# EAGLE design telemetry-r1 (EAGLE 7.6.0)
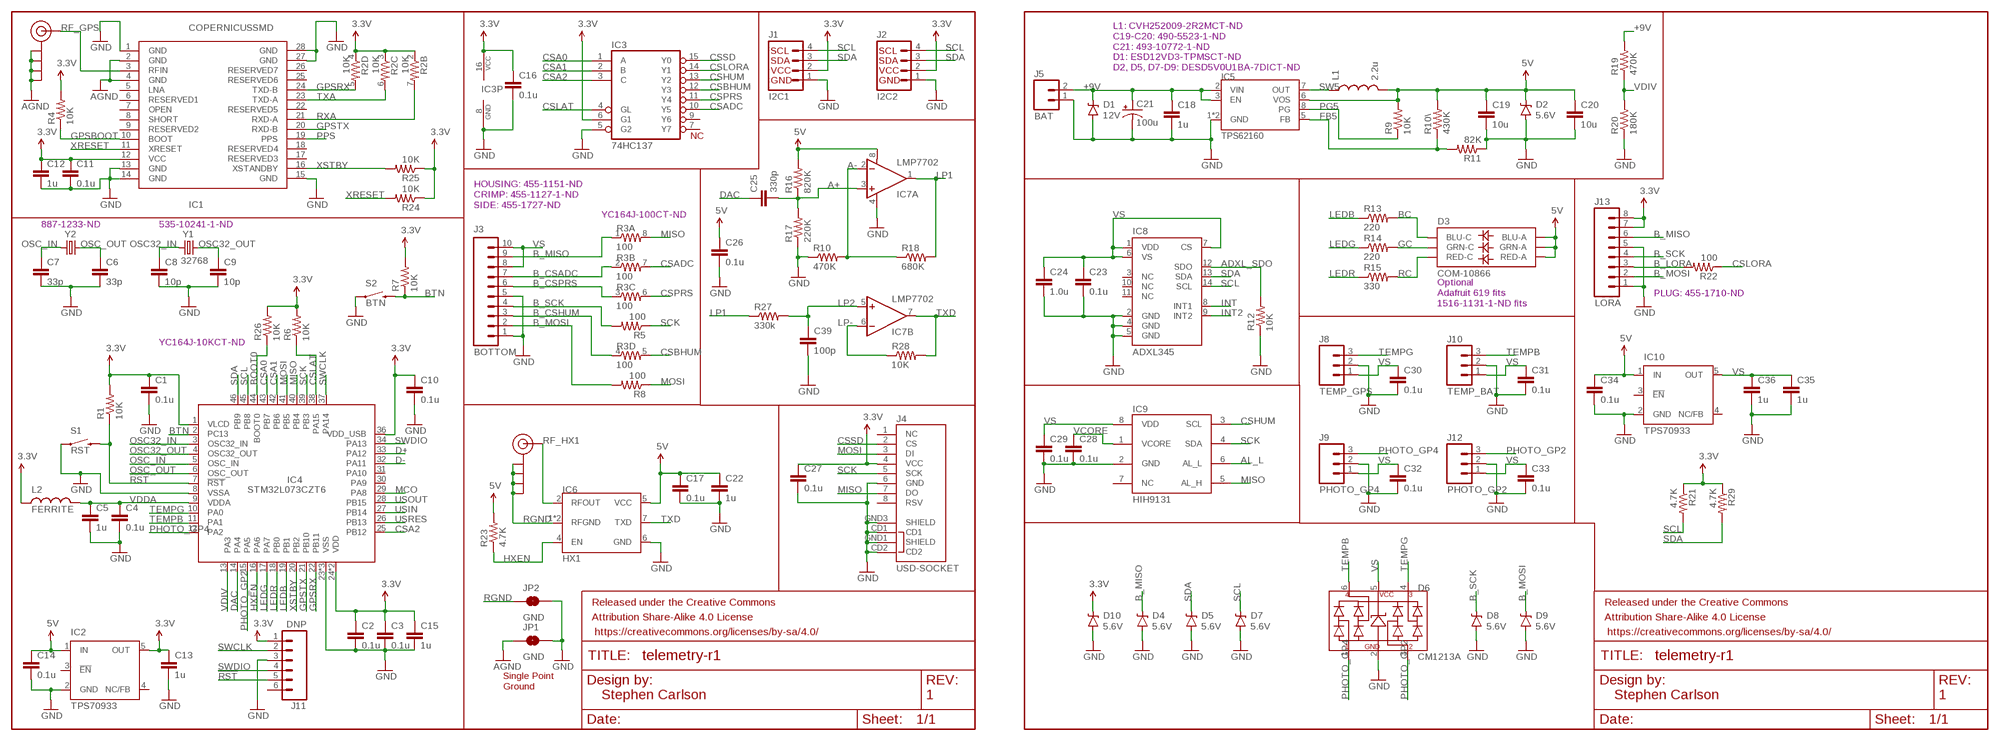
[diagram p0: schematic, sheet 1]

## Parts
C1  0.1u  CAP0805  [0805]
C2  0.1u  CAP0805  [0805]
C3  0.1u  CAP0805  [0805]
C4  0.1u  CAP0805  [0805]
C5  1u  CAP0805  [0805]
C6  33p  CAP0805  [0805]
C7  33p  CAP0805  [0805]
C8  10p  CAP0805  [0805]
C9  10p  CAP0805  [0805]
C10  0.1u  CAP0805  [0805]
C11  0.1u  CAP0805  [0805]
C12  1u  CAP0805  [0805]
C13  1u  CAP0805  [0805]
C14  0.1u  CAP0805  [0805]
C15  1u  CAP0805  [0805]
C16  0.1u  CAP0805  [0805]
C17  0.1u  CAP0805  [0805]
C18  1u  CAP0805  [0805]
C19  10u  CAP0805  [0805]
C20  10u  CAP0805  [0805]
C21  100u  CAP_POLPTH2  [CPOL-RADIAL-10UF-25V]
C22  1u  CAP0805  [0805]
C23  0.1u  CAP0805  [0805]
C24  1.0u  CAP0805  [0805]
C25  330p  CAP0805  [0805]
C26  0.1u  CAP0805  [0805]
C27  0.1u  CAP0805  [0805]
C28  0.1u  CAP0805  [0805]
C29  0.1u  CAP0805  [0805]
C30  0.1u  CAP0805  [0805]
C31  0.1u  CAP0805  [0805]
C32  0.1u  CAP0805  [0805]
C33  0.1u  CAP0805  [0805]
C34  0.1u  CAP0805  [0805]
C35  1u  CAP0805  [0805]
C36  1u  CAP0805  [0805]
C39  100p  CAP0805  [0805]
D1  12V  DIODE-ZENER5.6V  [SOD-323]
D2  5.6V  DIODE-ZENER5.6V  [SOD-323]
D3  COM-10866  LED-TRICOLOR-5050NO_IC  [LED-TRICOLOR-5050]
D4  5.6V  DIODE-ZENER5.6V  [SOD-323]
D5  5.6V  DIODE-ZENER5.6V  [SOD-323]
D6  CM1213A  [SC70-6L]
D7  5.6V  DIODE-ZENER5.6V  [SOD-323]
D8  5.6V  DIODE-ZENER5.6V  [SOD-323]
D9  5.6V  DIODE-ZENER5.6V  [SOD-323]
D10  5.6V  DIODE-ZENER5.6V  [SOD-323]
FRAME1  FRAME-LETTERNO_PACKAGE  [DUMMY]
FRAME2  FRAME-LETTERNO_PACKAGE  [DUMMY]
IC1  COPERNICUSSMD  [COPERNICUS]
IC2  TPS70933  TPS77033  [SOT23-DBV]
IC3  74HC137  74LS137PW  [TSSOP16]
IC4  STM32L073CZT6  STM32L07C  [TQFP48]
IC5  TPS62160  [MSOP8]
IC6  HX1  [HX1]
IC7  LMP7702  OPAMP-DUALU  [SO08]
IC8  ADXL345  [LGA14]
IC9  HIH9131  HIH6131  [SOIC8]
IC10  TPS70933  TPS77033  [SOT23-DBV]
J1  I2C1  I2C_STANDARD_NO_SILK  [1X04_NO_SILK]
J2  I2C2  I2C_STANDARD_NO_SILK  [1X04_NO_SILK]
J3  BOTTOM  M102MM  [1X10-2MM]
J4  USD-SOCKET  [MICROSD_1:1]
J5  BAT  M02PTH  [1X02]
J6  SMA_EDGE  [SMA-EDGE]
J7  SMA_EDGE  [SMA-EDGE]
J8  TEMP_GPS  M03JST-PTH  [JST-3-PTH]
J9  PHOTO_GP4  M03JST-PTH  [JST-3-PTH]
J10  TEMP_BAT  M03JST-PTH  [JST-3-PTH]
J11  DNP  M06LOCK  [1X06_LOCK]
J12  PHOTO_GP2  M03JST-PTH  [JST-3-PTH]
J13  LORA  1X08  [1X08-2MM]
JP1  GND  JUMPER-PAD-2-NC_BY_TRACE  [PAD-JUMPER-2-NC_BY_TRACE_YES_SILK]
JP2  GND  JUMPER-PAD-2-NC_BY_TRACE  [PAD-JUMPER-2-NC_BY_TRACE_YES_SILK]
L1  2.2u  INDUCTOR1008  [1008]
L2  FERRITE  INDUCTOR1206  [1206]
R1  10K  RESISTOR0805-RES  [0805]
R2  10K  RESISTOR-ARRAY0603-ARV  [0603-ARV]
R3  100  RESISTOR-ARRAY0603-ARV  [0603-ARV]
R4  10K  RESISTOR0805-RES  [0805]
R5  100  RESISTOR0805-RES  [0805]
R6  10K  RESISTOR0805-RES  [0805]
R7  10K  RESISTOR0805-RES  [0805]
R8  100  RESISTOR0805-RES  [0805]
R9  10K  RESISTOR0805-RES  [0805]
R10  470K  RESISTOR0805-RES  [0805]
R10\  430K  RESISTOR0805-RES  [0805]
R11  82K  RESISTOR0805-RES  [0805]
R12  10K  RESISTOR0805-RES  [0805]
R13  220  RESISTOR0805-RES  [0805]
R14  220  RESISTOR0805-RES  [0805]
R15  330  RESISTOR0805-RES  [0805]
R16  820K  RESISTOR0805-RES  [0805]
R17  220K  RESISTOR0805-RES  [0805]
R18  680K  RESISTOR0805-RES  [0805]
R19  470K  RESISTOR0805-RES  [0805]
R20  180K  RESISTOR0805-RES  [0805]
R21  4.7K  RESISTOR0805-RES  [0805]
R22  100  RESISTOR0805-RES  [0805]
R23  4.7K  RESISTOR0805-RES  [0805]
R24  10K  RESISTOR0805-RES  [0805]
R25  10K  RESISTOR0805-RES  [0805]
R26  10K  RESISTOR0805-RES  [0805]
R27  330k  RESISTOR0805-RES  [0805]
R28  10K  RESISTOR0805-RES  [0805]
R29  4.7K  RESISTOR0805-RES  [0805]
S1  RST  SWITCH  [TACTILE-PTH-THIN]
S2  BTN  SWITCH  [TACTILE-PTH-THIN]
Y1  32768  CRYSTAL  [ABS25]
Y2  8M  CRYSTALSMD  [HC49UP]

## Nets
3.3V: C1.1 C2.1 C3.1 C10.1 C11.1 C12.1 C13.1 C15.1 C16.1 C27.1 D10.C IC1.12(VCC) IC2.5(OUT) IC3.6(G1) IC3.16(VCC) IC4.1(VLCD) IC4.24(VDD) IC4.36(VDD_USB) IC4.48(VDD) J1.2 J2.2 J4.4(VCC) J11.1 J13.7 J13.8 L2.1 R1.2 R2.2 R2.3 R2.4 R4.2 R6.2 R7.2 R21.1 R24.1 R25.1 R26.2 R29.1
5V: C14.1 C17.1 C19.1 C20.1 C22.1 C26.1 C34.1 D2.C D3.1(GRN-A) D3.2(RED-A) D3.3(BLU-A) IC2.1(IN) IC5.6(VOS) IC6.5(VCC) IC7.8(A:V+) IC10.1(IN) L1.2 R9.2 R10\.2 R16.2 R23.2
!RST!: IC4.7(!RST!) J11.5 R1.1 S1.2
+9V: C18.1 C21.1(+) D1.C IC5.2(VIN) IC5.3(EN) J5.2 R19.2
A+: C25.2 IC7.3(A:+IN) R16.1 R17.2
A-: IC7.2(A:-IN) R10.2 R18.1
ADXL_SDO: IC8.12(SDO) R12.2
AGND: IC1.2(GND) IC1.4(GND) J7.GND@0(GND) J7.GND@1(GND) J7.GND@2(GND) J7.GND@3(GND) JP1.1
AL_L: IC9.6(AL_L)
B_CSADC: J3.7 R3.2
B_CSHUM: J3.3 R3.4
B_CSPRS: J3.6 R3.3
B_LORA: J13.3 R22.2
B_MISO: D4.C J3.9 J13.6 R3.1
B_MOSI: D9.C J3.2 J13.2 R8.2
B_SCK: D8.C J3.4 J13.4 R5.2
BC: D3.4(BLU-C) R13.2
BOOT0: IC4.44(BOOT0) R26.1
BTN: IC4.2(PC13) R7.1 S2.2
CSA0: IC3.1(A) IC4.43(PB7)
CSA1: IC3.2(B) IC4.42(PB6)
CSA2: IC3.3(C) IC4.25(PB12)
CSADC: IC3.10(Y5) R3.7
CSBHUM: IC3.12(Y3) R3.5
CSHUM: IC3.13(Y2) IC9.3(SCL)
CSLAT: IC3.4(GL) IC4.38(PA15) R6.1
CSLORA: IC3.14(Y1) R22.1
CSPRS: IC3.11(Y4) R3.6
CSSD: IC3.15(Y0) J4.2(CS)
D+: IC4.33(PA12)
D-: IC4.32(PA11)
DAC: C25.1 IC4.14(PA4)
FB5: IC5.5(FB) R10\.1 R11.2
GC: D3.6(GRN-C) R14.2
GND: C1.2 C2.2 C3.2 C4.2 C5.2 C6.2 C7.2 C8.2 C9.2 C10.2 C11.2 C12.2 C13.2 C14.2 C15.2 C16.2 C17.2 C18.2 C19.2 C20.2 C21.2(-) C22.2 C23.2 C24.2 C26.2 C27.2 C28.2 C29.2 C30.2 C31.2 C32.2 C33.2 C34.2 C35.2 C36.2 C39.2 D1.A D2.A D4.A D5.A D6.2(GND) D7.A D8.A D9.A D10.A IC1.1(GND) IC1.13(GND) IC1.14(GND) IC1.15(GND) IC1.27(GND) IC1.28(GND) IC2.2(GND) IC3.5(G2) IC3.8(GND) IC4.8(VSSA) IC4.23(VSS) IC4.35(VSS) IC4.47(VSS) IC5.1(GND) IC5.4(GND) IC6.6(GND) IC7.4(A:V-) IC8.2(GND) IC8.4(GND) IC8.5(GND) IC9.2(GND) IC10.2(GND) J1.1 J2.1 J3.1 J3.5 J4.6(GND) J4.CD1 J4.CD2 J4.GND1(SHIELD) J4.GND3(SHIELD) J5.1 J8.2 J9.2 J10.2 J11.3 J12.2 J13.1 J13.5 JP1.2 JP2.2 R10.1 R11.1 R12.1 R17.1 R20.1 S1.1 S2.1
GPSBOOT: IC1.10(BOOT) R4.1
GPSRX: IC1.24(TXD-B) IC4.22(PB11) R2.5
GPSTX: IC1.20(RXD-B) IC4.21(PB10)
HXEN: IC4.16(PA6) IC6.4(EN) R23.1
INT: IC8.8(INT1)
INT2: IC8.9(INT2)
LEDB: IC4.19(PB1) R13.1
LEDG: IC4.17(PA7) R14.1
LEDR: IC4.18(PB0) R15.1
LP1: IC7.1(A:OUT) R18.2 R27.1
LP2: C39.1 IC7.5(B:+IN) R27.2
LP-: IC7.6(B:-IN) R28.1
MCO: IC4.29(PA8)
MISO: IC4.40(PB4) IC9.5(AL_H) J4.7(DO) R3.8
MOSI: IC4.41(PB5) J4.3(DI) R8.1
OSC32_IN: C8.1 IC4.3(OSC32_IN) Y1.1
OSC32_OUT: C9.1 IC4.4(OSC32_OUT) Y1.4
OSC_IN: C7.1 IC4.5(OSC_IN) Y2.1
OSC_OUT: C6.1 IC4.6(OSC_OUT) Y2.2
PG5: IC5.8(PG) R9.1
PHOTO_GP2: D6.3(CH2) IC4.15(PA5) J12.3
PHOTO_GP4: D6.1(CH1) IC4.12(PA2) J9.3
PPS: IC1.19(PPS)
RC: D3.5(RED-C) R15.2
RF_GPS: IC1.3(RFIN) J7.SIG(SIGNAL)
RF_HX1: IC6.2(RFOUT) J6.SIG(SIGNAL)
RGND: IC6.1(RFGND) IC6.3(RFGND) J6.GND@0(GND) J6.GND@1(GND) J6.GND@2(GND) J6.GND@3(GND) JP2.1
RXA: IC1.21(RXD-A) R2.7
SCK: IC4.39(PB3) IC9.4(SDA) J4.5(SCK) R5.1
SCL: D7.C IC4.45(PB8) IC8.14(SCL) J1.4 J2.4 R21.2
SDA: D5.C IC4.46(PB9) IC8.13(SDA) J1.3 J2.3 R29.2
SW5: IC5.7(OUT) L1.1
SWCLK: IC4.37(PA14) J11.2
SWDIO: IC4.34(PA13) J11.4
TEMPB: D6.6(CH4) IC4.11(PA1) J10.3
TEMPG: D6.4(CH3) IC4.10(PA0) J8.3
TXA: IC1.23(TXD-A) R2.6
TXD: IC6.7(TXD) IC7.7(B:OUT) R28.2
USIN: IC4.27(PB14)
USOUT: IC4.28(PB15)
USRES: IC4.26(PB13)
VCORE: C28.1 IC9.1(VCORE)
VDDA: C4.1 C5.1 IC4.9(VDDA) L2.2
VDIV: IC4.13(PA3) R19.1 R20.2
VS: C23.1 C24.1 C29.1 C30.1 C31.1 C32.1 C33.1 C35.1 C36.1 D6.5(VCC) IC8.1(VDD) IC8.6(VS) IC8.7(CS) IC9.8(VDD) IC10.5(OUT) J3.8 J3.10 J8.1 J9.1 J10.1 J12.1
XRESET: IC1.11(XRESET) R24.2
XSTBY: IC1.16(XSTANDBY) IC4.20(PB2) R25.2
Unconnected: IC1.5(LNA) IC1.6(RESERVED1) IC1.7(OPEN) IC1.8(SHORT) IC1.9(RESERVED2) IC1.17(RESERVED3) IC1.18(RESERVED4) IC1.22(RESERVED5) IC1.25(RESERVED6) IC1.26(RESERVED7) IC2.3(!EN) IC2.4(NC/FB) IC3.7(Y7) IC3.9(Y6) IC4.30(PA9) IC4.31(PA10) IC8.3(NC) IC8.10(NC) IC8.11(NC) IC9.7(NC) IC10.3(!EN) IC10.4(NC/FB) J4.1(NC) J4.8(RSV) J11.6 R2.1 R2.8

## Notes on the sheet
- L1: CVH252009-2R2MCT-ND
  C19-C20: 490-5523-1-ND
  C21: 493-10772-1-ND
  D1: ESD12VD3-TPMSCT-ND
  D2, D5, D7-D9: DESD5V0U1BA-7DICT-ND
- NC
- HOUSING: 455-1151-ND
  CRIMP: 455-1127-1-ND
  SIDE: 455-1727-ND
- YC164J-100CT-ND
- 887-1233-ND | 535-10241-1-ND
- PLUG: 455-1710-ND
- Optional
  Adafruit 619 fits
  1516-1131-1-ND fits
- YC164J-10KCT-ND
- Single Point
  Ground
- Stephen Carlson | 1 | Stephen Carlson | 1

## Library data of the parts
C1-C20 C22-C36 C39 = SparkFun-Passives:CAP: Capacitor
C21 = SparkFun-Passives:CAP_POL: Capacitor Polarized
D1 = SparkFun-DiscreteSemi:DIODE-ZENER: Zener Diode; PROD_ID: DIO-12442; VALUE: 5.6V
D2 D4 D5 D7-D10 = SparkFun-DiscreteSemi:DIODE-ZENER: Zener Diode; PROD_ID: DIO-12442
D3 = SparkFun-LED:LED-TRICOLOR-5050
D6 = HAB:CM1213A: CM1213A CM1213A 4-channel ESD protection device
FRAME1 FRAME2 = SparkFun-Aesthetics:FRAME-LETTER: Schematic Frame; DESIGNER: Nobody; VERSION: v01
IC1 = SparkFun-RF:COPERNICUS: Copernicus II GPS- Trimble recommended layout and paste layer. Footprint production proven. Spark Fun Electronics SKU : GPS-07951
IC2 IC10 = texas:TPS770*: ULTRALOW-POWER 50-mA LOW-DROPOUT LINEAR REGULATORS 50-mA Low-Dropout Regulator Source: http://focus.ti.com/lit/ds/symlink/tps77001.pdf; MF: TEXAS INSTRUMENTS; MPN: TPS77033DBVT; OC_FARNELL: 8461570; OC_NEWARK: 77C1187
IC3 = HAB:74*137: 3-line to 8-line DECODER/DEMULTIPLEXER, address LATCH
IC4 = stm32xx:STM32L07*C: STM32L07XC STM32L07X series in LQFP-48 package
IC5 = HAB:TPS62160: TPS62160 Adjustable switch-mode D-CAP2 regulator
IC6 = HAB:HX1: Radiometrix HX1 High-power VHF Narrow Band 300 mW Transmitter
IC7 = SparkFun-AnalogIC:OPAMP-DUAL: Generic op-amp footprint
IC8 = SparkFun-Sensors:ADXL345: 3-axis SPI/I2C 2/4/8/16g accelerometer
IC9 = SparkFun-AnalogIC:HIH6131
J1 J2 = SparkFun-Connectors:I2C_STANDARD: SparkFun has standardized on a pinout for all I2C based sensor breakouts. This pinout allows I2C boards to be plugged directly into the headers on Arduino Uno compatible boards, and to be daisy chained easily.
J3 = SparkFun-Connectors:M10: Header 10 Standard 10-pin 0.1" header. Use with straight break away headers (SKU : PRT-00116), right angle break away headers (PRT-00553), swiss pins (PRT-00743), machine pins (PRT-00117), and female headers (PRT-00115).
J4 = SparkFun-Connectors:USD-SOCKET: microSD Socket Push-push type uSD socket. Schematic element and footprint production proven. Spark Fun Electronics SKU : PRT-00127. tDoc lines correctly indicate media card edge positions when inserting (unlocked, locked, depressed). NOTE: CD1 and CD2 are connected internally; PROD_ID: CONN-07820
J5 = SparkFun-Connectors:M02: Standard 2-pin 0.1" header. Use with
J6 J7 = SparkFun-Connectors:SMA_EDGE: SMA Antenna Connector End launch SMA connector. The paste layer has been removed so that the connector can be hand soldered onto the board after reflow.
J8-J10 J12 = SparkFun-Connectors:M03: Header 3 Standard 3-pin 0.1" header. Use with straight break away headers (SKU : PRT-00116), right angle break away headers (PRT-00553), swiss pins (PRT-00743), machine pins (PRT-00117), and female headers (PRT-00115). Molex polarized connector foot print use with SKU : PRT-08232 with associated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; SKU: PRT-09915
J11 = SparkFun-Connectors:M06: Header 6 Standard 6-pin 0.1" header. Use with straight break away headers (SKU : PRT-00116), right angle break away headers (PRT-00553), swiss pins (PRT-00743), machine pins (PRT-00117), and female headers (PRT-00115). Molex polarized connector foot print use with SKU : PRT-08094 with associated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
J13 = HAB:1X08: 1X08 1x8 header
JP1 JP2 = SparkFun-Passives:JUMPER-PAD-2-NC_BY_TRACE
L1 L2 = HAB:INDUCTOR: INDUCTOR
R1 R4-R10 R10\ R11-R29 = SparkFun-Passives:RESISTOR: Resistor
R2 R3 = SparkFun-Passives:RESISTOR-ARRAY: Array Chip Resistor Source: RS Component / Phycomp
S1 S2 = HAB:SWITCH: SWITCH
Y1 = HAB:CRYSTAL: CRYSTAL
Y2 = SparkFun-FreqCtrl:CRYSTAL: Various standard crystals. Proven footprints.

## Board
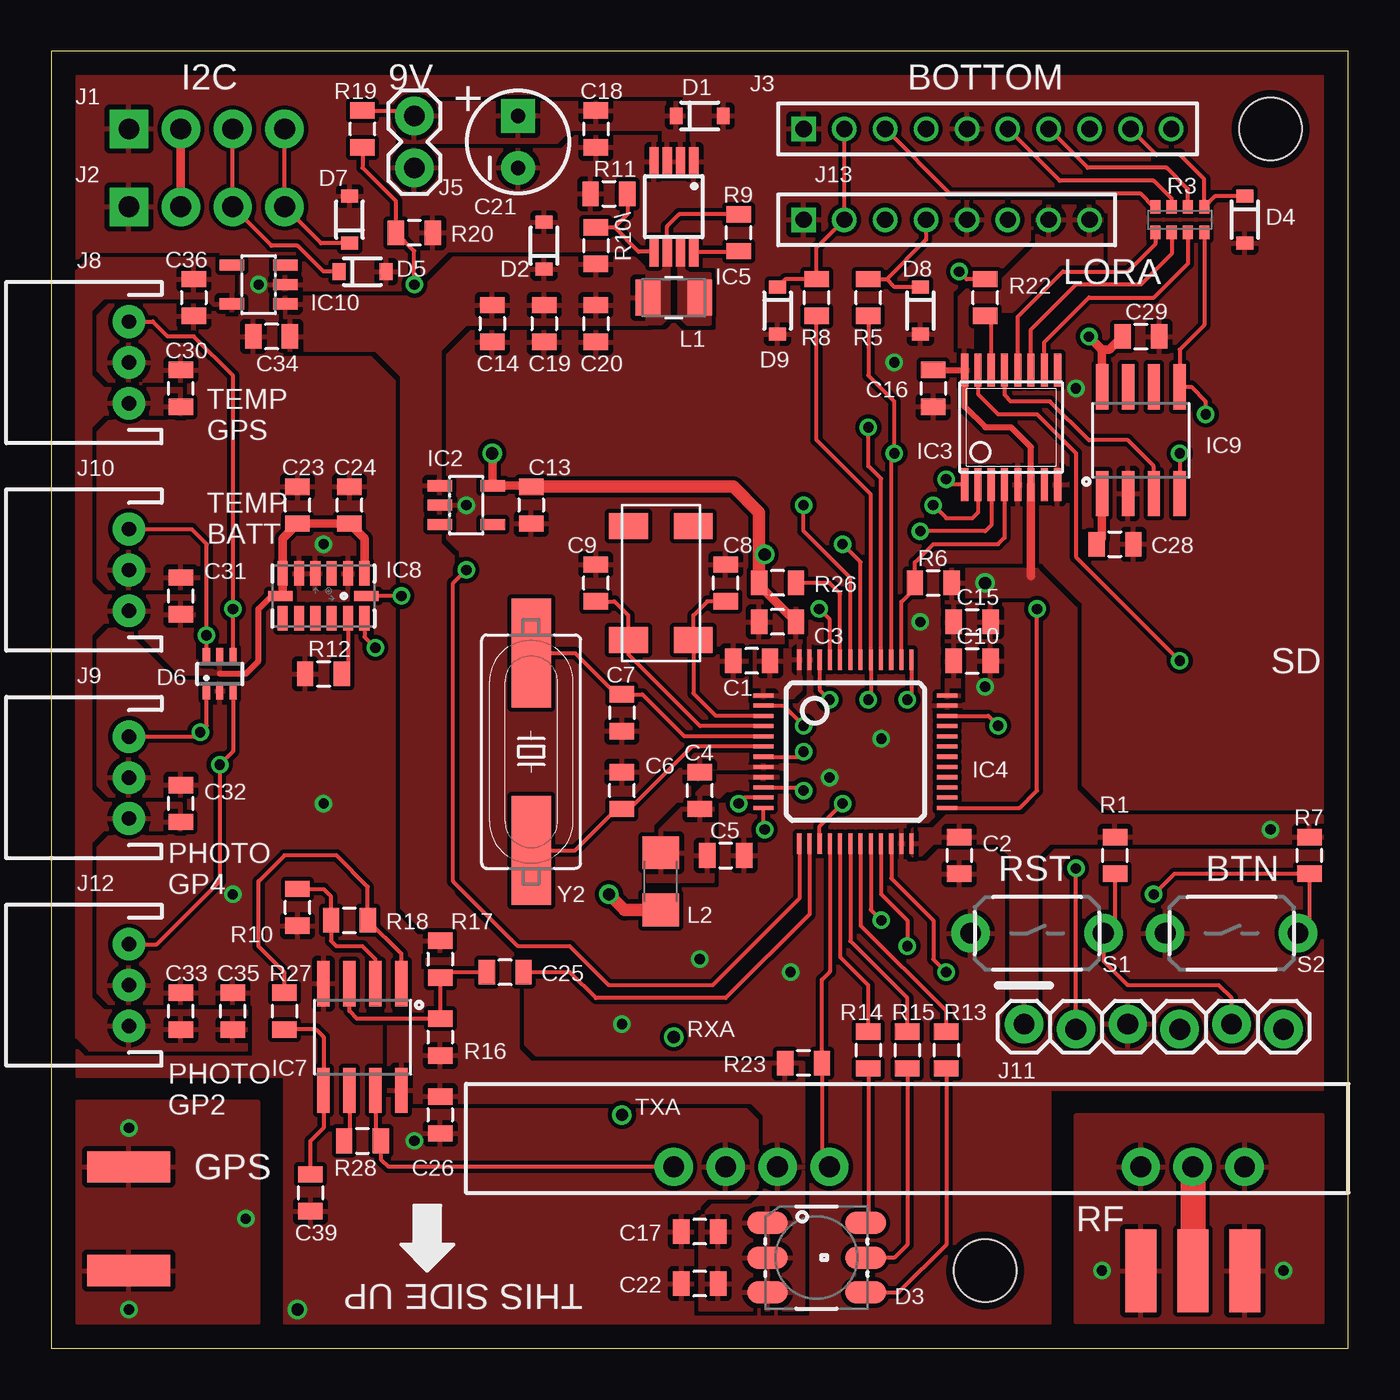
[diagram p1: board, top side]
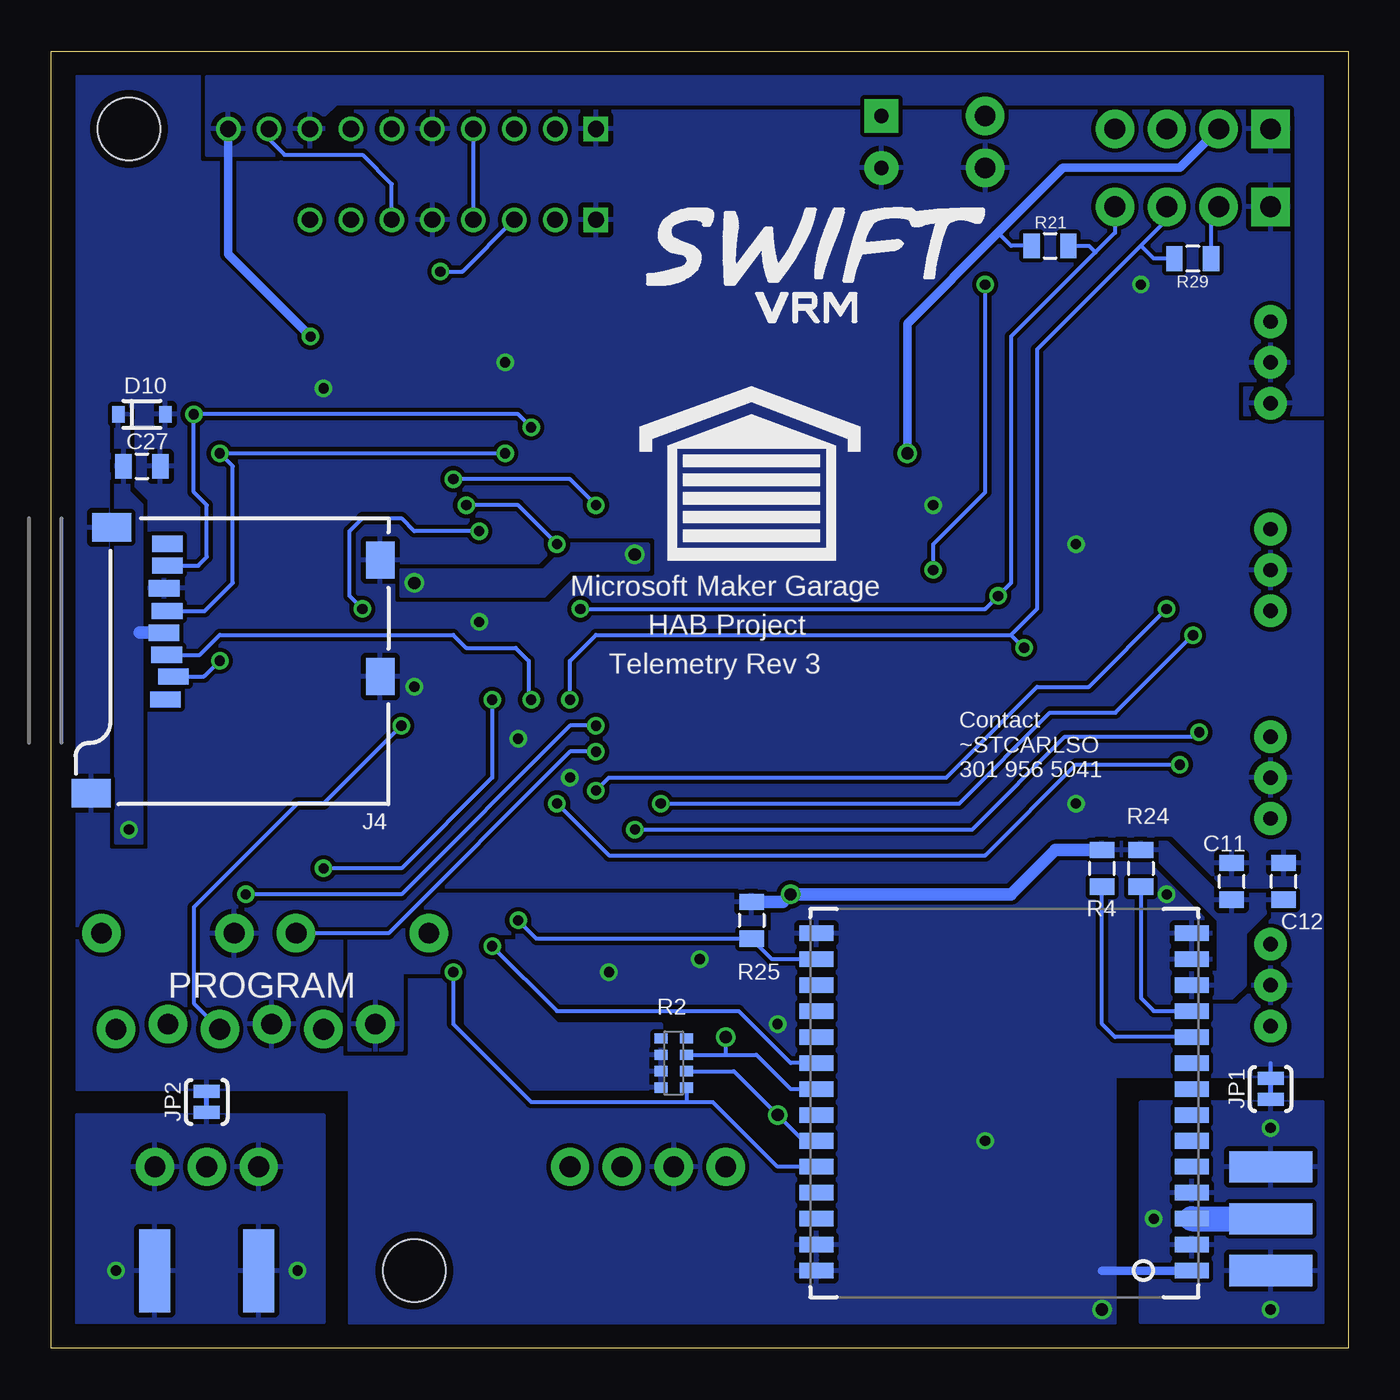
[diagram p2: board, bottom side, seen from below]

Size 63.5 x 63.5 mm. Coordinates in mm from the lower left corner, seen from the top.
Outline: 0,0 63.5,0 63.5,63.5 0,63.5 0,0
Copper layers (1*16): Top 0.0356mm / dielectric 1.5011mm / Bottom 0.0356mm
Design rules "LaenPCBOrder *": minimum track width 6mil, minimum drill 13mil, track to track 8mil, track to pad 8mil, pad to pad 8mil, via to via 8mil, smd to smd 6mil, copper to edge 15mil, drill to drill 6mil, minimum pad ring 7mil, minimum via ring 7mil, stop-mask expansion 3mil, vias tented up to drill 0mil, thermal gap 10mil
Holes 3.05 mm at 45.72,3.81 59.69,59.69

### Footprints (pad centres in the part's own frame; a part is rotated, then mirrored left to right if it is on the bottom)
0805 = smd 0.8 x 1.2: 1 -0.9,0; 2 0.9,0
CPOL-RADIAL-10UF-25V = drill 0.7 pad 1.651 square: 1 1.27,0 | drill 0.7 pad 1.651: 2 -1.27,0
SOD-323 = smd 0.63 x 0.83: A 1.15,0; C -1.15,0
LED-TRICOLOR-5050 = smd 2 x 1.1: 1 -2.4,1.7; 2 -2.4,0; 3 -2.4,-1.7; 4 2.4,-1.7; 5 2.4,0; 6 2.4,1.7
SC70-6L = smd 0.35 x 0.8: 1 -0.65,-0.85; 2 0,-0.85; 3 0.65,-0.85; 4 0.65,0.85; 5 0,0.85; 6 -0.65,0.85
COPERNICUS = smd 0.762 x 1.651: 1 0,-18.364; 2 1.27,-18.364; 3 2.54,-18.364; 4 3.81,-18.364; 5 5.08,-18.364; 6 6.35,-18.364; 7 7.62,-18.364; 8 8.89,-18.364; 9 10.16,-18.364; 10 11.43,-18.364; 11 12.7,-18.364; 12 13.97,-18.364; 13 15.24,-18.364; 14 16.51,-18.364; 15 16.51,0; 16 15.24,0; 17 13.97,0; 18 12.7,0; 19 11.43,0; 20 10.16,0; 21 8.89,0; 22 7.62,0; 23 6.35,0; 24 5.08,0; 25 3.81,0; 26 2.54,0; 27 1.27,0; 28 0,0
SOT23-DBV = smd 0.55 x 1.2: 1 -0.95,-1.3; 2 0,-1.3; 3 0.95,-1.3; 4 0.95,1.3; 5 -0.95,1.3
TSSOP16 = smd 0.35 x 1.6: 1 -2.275,-2.8; 2 -1.625,-2.8; 3 -0.975,-2.8; 4 -0.325,-2.8; 5 0.325,-2.8; 6 0.975,-2.8; 7 1.625,-2.8; 8 2.275,-2.8; 9 2.275,2.8; 10 1.625,2.8; 11 0.975,2.8; 12 0.325,2.8; 13 -0.325,2.8; 14 -0.975,2.8; 15 -1.625,2.8; 16 -2.275,2.8
TQFP48 = smd 0.2 x 1: 1 -2.75,-4.5; 2 -2.25,-4.5; 3 -1.75,-4.5; 4 -1.25,-4.5; 5 -0.75,-4.5; 6 -0.25,-4.5; 7 0.25,-4.5; 8 0.75,-4.5; 9 1.25,-4.5; 10 1.75,-4.5; 11 2.25,-4.5; 12 2.75,-4.5; 25 2.75,4.5; 26 2.25,4.5; 27 1.75,4.5; 28 1.25,4.5; 29 0.75,4.5; 30 0.25,4.5; 31 -0.25,4.5; 32 -0.75,4.5; 33 -1.25,4.5; 34 -1.75,4.5; 35 -2.25,4.5; 36 -2.75,4.5 | smd 1 x 0.2: 13 4.5,-2.75; 14 4.5,-2.25; 15 4.5,-1.75; 16 4.5,-1.25; 17 4.5,-0.75; 18 4.5,-0.25; 19 4.5,0.25; 20 4.5,0.75; 21 4.5,1.25; 22 4.5,1.75; 23 4.5,2.25; 24 4.5,2.75; 37 -4.5,2.75; 38 -4.5,2.25; 39 -4.5,1.75; 40 -4.5,1.25; 41 -4.5,0.75; 42 -4.5,0.25; 43 -4.5,-0.25; 44 -4.5,-0.75; 45 -4.5,-1.25; 46 -4.5,-1.75; 47 -4.5,-2.25; 48 -4.5,-2.75
MSOP8 = smd 0.45 x 1.45: 1 -0.975,-2.2; 2 -0.325,-2.2; 3 0.325,-2.2; 4 0.975,-2.2; 5 0.975,2.2; 6 0.325,2.2; 7 -0.325,2.2; 8 -0.975,2.2
HX1 = drill 1.016 pad 1.88: 1 0,0; 2 2.54,0; 3 5.08,0; 4 20.32,0; 5 22.86,0; 6 25.4,0; 7 27.94,0
SO08 = smd 0.61 x 2.21: 1 -1.905,-2.616; 2 -0.635,-2.616; 3 0.635,-2.616; 4 1.905,-2.616; 5 1.905,2.616; 6 0.635,2.616; 7 -0.635,2.616; 8 -1.905,2.616
LGA14 = smd 0.5 x 1.2: 1 2,1.1; 2 1.2,1.1; 3 0.4,1.1; 4 -0.4,1.1; 5 -1.2,1.1; 6 -2,1.1; 8 -2,-1.1; 9 -1.2,-1.1; 10 -0.4,-1.1; 11 0.4,-1.1; 12 1.2,-1.1; 13 2,-1.1 | smd 1.2 x 0.5: 7 -2.1,0; 14 2.1,0
SOIC8 = smd 0.61 x 2.21: 1 -1.905,-2.616; 2 -0.635,-2.616; 3 0.635,-2.616; 4 1.905,-2.616; 5 1.905,2.616; 6 0.635,2.616; 7 -0.635,2.616; 8 -1.905,2.616
1X04_NO_SILK = drill 1.016 pad 1.88 square: 1 0,0 | drill 1.016 pad 1.88: 2 2.54,0; 3 5.08,0; 4 7.62,0
1X10-2MM = drill 0.8 square: 1 0,0 | drill 0.8: 2 2,0; 3 4,0; 4 6,0; 5 8,0; 6 10,0; 7 12,0; 8 14,0; 9 16,0; 10 18,0
MICROSD_1:1 = smd 0.8 x 1.5: 1 5.096,10.919; 2 6.218,10.519; 3 7.274,10.853; 4 8.367,10.982; 5 9.421,10.828; 6 10.539,10.973; 7 11.648,10.819; 8 12.721,10.819 | smd 1.8 x 1.4: CD1 11.92,0.4; CD2 6.22,0.4 | smd 1.4 x 1.9: GND1 0.497,14.55; GND3 13.52,13.55
1X02 = drill 1.016 pad 1.88: 1 0,0; 2 2.54,0
SMA-EDGE = smd 1.524 x 4.064: GND@0 0,0; GND@1 5.08,0; SIG 2.54,0 | smd 1.524 x 4.064 bottom: GND@2 0,0; GND@3 5.08,0
JST-3-PTH = drill 0.7 pad 1.6: 1 -2,0; 2 0,0; 3 2,0
1X06_LOCK = drill 1.016 pad 1.88: 1 0,0; 2 2.54,-0.254; 3 5.08,0; 4 7.62,-0.254; 5 10.16,0; 6 12.7,-0.254
1X08-2MM = drill 0.8 square: 1 0,0 | drill 0.8: 2 2,0; 3 4,0; 4 6,0; 5 8,0; 6 10,0; 7 12,0; 8 14,0
PAD-JUMPER-2-NC_BY_TRACE_YES_SILK = smd 0.635 x 1.27: 1 -0.508,0; 2 0.508,0
1008 = smd 1.753 x 1.219: 1 0,1.27; 2 0,-1.27
1206 = smd 1.6 x 1.8: 1 -1.4,0; 2 1.4,0
0603-ARV = smd 0.5 x 0.65: 1 -1.2,-0.625; 2 -0.4,-0.625; 3 0.4,-0.625; 4 1.2,-0.625; 5 1.2,0.625; 6 0.4,0.625; 7 -0.4,0.625; 8 -1.2,0.625
TACTILE-PTH-THIN = drill 1.016 pad 1.88: 1 -3.251,0; 2 3.251,0
ABS25 = smd 1.27 x 1.905: 1 -2.794,-1.587; 2 2.794,-1.587; 3 2.794,1.587; 4 -2.794,1.587
HC49UP = smd 5.334 x 1.93: 1 -4.826,0; 2 4.826,0

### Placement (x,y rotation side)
C1  34.29,33.66 180 top
C2  44.45,24.13 270 top
C3  35.56,35.56 180 top
C4  31.75,27.3 90 top
C5  33.02,24.13 0 top
C6  27.94,27.3 90 top
C7  27.94,31.11 270 top
C8  33.02,37.47 90 top
C9  26.67,37.47 90 top
C10  45.09,33.66 0 top
C11  5.71,22.86 90 bottom
C12  3.17,22.86 90 bottom
C13  23.5,41.27 270 top
C14  21.59,50.16 270 top
C15  45.09,35.56 0 top
C16  43.18,46.99 270 top
C17  31.75,5.71 180 top
C18  26.67,59.69 270 top
C19  24.13,50.16 270 top
C20  26.67,50.16 270 top
C21  22.86,59.05 90 top
C22  31.75,3.17 180 top
C23  12.06,41.27 90 top
C24  14.61,41.27 90 top
C25  22.23,18.41 180 top
C26  19.05,11.43 270 top
C27  59.05,43.18 0 bottom
C28  52.07,39.37 0 top
C29  53.34,49.53 0 top
C30  6.35,46.99 90 top
C31  6.35,36.83 90 top
C32  6.35,26.67 90 top
C33  6.35,16.51 90 top
C34  10.79,49.53 180 top
C35  8.89,16.51 90 top
C36  6.99,51.44 270 top
C39  12.7,7.62 270 top
D1  31.75,60.33 0 top
D2  24.13,53.98 90 top
D3  37.47,4.45 0 top
D4  58.42,55.24 270 top
D5  15.24,52.7 0 top
D6  8.26,33.02 0 top
D7  14.61,55.24 90 top
D8  42.55,50.8 270 top
D9  35.56,50.8 270 top
D10  59.05,45.72 0 bottom
FRAME1  0,64.77 0 top
FRAME2  1.27,64.77 0 top
IC1  26.04,3.81 90 bottom
IC2  20.32,41.27 270 top
IC3  46.99,45.09 0 top
IC4  39.37,29.21 270 top
IC5  30.48,55.88 180 top
IC6  58.42,8.89 180 top
IC7  15.24,15.24 180 top
IC8  13.34,36.83 0 top
IC9  53.34,44.45 0 top
IC10  10.16,52.07 90 top
J1  3.81,59.69 0 top
J2  3.81,55.88 0 top
J3  36.83,59.69 0 top
J4  46.99,26.67 90 bottom
J5  17.78,57.78 90 top
J6  53.34,3.81 0 top
J7  3.81,3.81 90 bottom
J8  3.81,48.26 90 top
J9  3.81,27.94 90 top
J10  3.81,38.1 90 top
J11  47.62,15.88 0 top
J12  3.81,17.78 90 top
J13  36.83,55.24 0 top
JP1  3.81,12.7 90 bottom
JP2  55.88,12.06 90 bottom
L1  30.48,51.44 270 top
L2  29.84,22.86 90 top
R1  52.07,24.13 90 top
R2  33.02,13.97 270 bottom
R3  55.24,55.24 180 top
R4  12.06,23.5 90 bottom
R5  40.01,51.44 90 top
R6  43.18,37.47 0 top
R7  61.59,24.13 90 top
R8  37.47,51.44 90 top
R9  33.66,54.61 90 top
R10  12.06,21.59 90 top
R10\  26.67,53.98 270 top
R11  27.3,56.52 0 top
R12  13.34,33.02 0 top
R13  43.81,14.61 270 top
R14  40.01,14.61 270 top
R15  41.91,14.61 270 top
R16  19.05,15.24 270 top
R17  19.05,19.05 270 top
R18  14.61,20.95 0 top
R19  15.24,59.69 90 top
R20  17.78,54.61 180 top
R21  14.61,53.98 0 bottom
R22  45.72,51.44 90 top
R23  36.83,13.97 180 top
R24  10.16,23.5 270 bottom
R25  29.21,20.95 270 bottom
R26  35.56,37.47 180 top
R27  11.43,16.51 270 top
R28  15.24,10.16 0 top
R29  7.62,53.34 180 bottom
S1  48.26,20.32 0 top
S2  57.78,20.32 0 top
U$2  [GARAGE]  29.21,41.91 0 bottom
U$5  [SWIFT]  27.3,52.7 0 bottom
Y1  29.84,37.47 90 top
Y2  23.5,29.21 270 top

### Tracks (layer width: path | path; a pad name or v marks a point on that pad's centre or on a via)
3.3V  (via drill 0.5, 0.6)
  Top 0.305: C16.1 IC3.16 44.72,46.09 45.72,45.09 46.99,45.09 47.97,44.11 IC3.6
  Top 0.406: J2.2 J1.2 | R26.2 34.66,37.36 C3.1 | IC3.6 47.97,37.8 | C13.1 23.45,42.23 IC2.5 21.62,43.78 v21.59,43.81
  Top 0.61: L2.1 28.07,21.46 v27.3,22.23 | R26.2 34.66,38.86 | 34.66,38.86 34.66,40.91 33.39,42.17 C13.1 | v34.92,38.86 34.66,38.86
  Bottom 0.203: R21.1 16.51,53.98 17.14,54.61 | R29.1 6.72,55.51 J2.2
  Bottom 0.406: v21.59,43.81 21.59,50.16 17.14,54.61 13.97,57.78 8.26,57.78 J1.2
  Bottom 0.61: R4.2 14.34,24.39 16.51,22.23 v27.3,22.23 27.68,21.86 R25.1 | J4.4 59.17,35.04
  other vias: 59.69,25.4 45.72,37.47
  pour Top (isolate 0.203, rank 2): 34.42,34.16 34.42,31.88 36.32,31.88 36.7,32.26 36.7,36.2 36.2,36.2 36.2,34.16
  pour Bottom (rank 2): 3.17,22.23 5.08,20.32 5.08,17.78 5.71,17.14 8.26,17.14 8.26,18.41 6.35,18.41 6.35,20.95 9.53,24.13 12.7,24.13 12.7,24.77 8.89,24.77 6.35,22.23
  pour Top (isolate 0.203, rank 2): 42.16,25.4 42.16,24.13 42.55,24.13 43.18,24.77 46.35,24.77 46.99,24.13 46.99,15.88 48.26,15.88 48.26,24.13 48.9,24.77 62.23,24.77 62.23,26.04 51.44,26.04 50.16,27.3 50.16,36.2 48.26,38.1 43.81,38.1 43.81,31.75 44.45,31.75 44.45,36.83 48.26,36.83 48.26,26.67 47.62,26.04 43.81,26.04 43.18,25.4
  pour Bottom (isolate 0.203, rank 3): 60.33,24.77 59.05,24.77 59.05,41.27 59.69,41.91 59.69,45.72 60.33,45.72
  pour Top (isolate 0.203, rank 3): 48.26,55.88 48.26,53.98 46.35,52.07 45.09,52.07 44.45,51.44 44.45,47.62 45.09,47.62 45.09,50.8 47.62,50.8 49.53,52.7 50.8,52.7 51.44,53.34 51.44,55.88
  pour Bottom (isolate 0.203, rank 2): 33.66,15.88 33.66,12.7 40.01,12.7 43.18,15.88 43.18,18.41 46.35,18.41 46.35,14.61 48.9,14.61 48.9,20.32 46.99,20.32 45.09,22.23 28.57,22.23 28.57,20.32 41.91,20.32 41.91,19.05 38.73,15.88
  pour Bottom (isolate 0.203, rank 2): 34.29,39.37 34.29,38.1 38.1,38.1 39.37,36.83 46.35,36.83 46.35,38.1 39.37,38.1 38.1,39.37
5V
  Top 0.203: R9.2 30.75,55.51 30.16,54.92 IC5.6
  pour Top (isolate 0.203, rank 2, no thermals): 30.23,53.98 30.23,50.55 29.84,50.16 29.21,50.16 29.21,52.7 29.84,52.7 29.84,53.98
  pour Top (isolate 0.203, rank 2): 29.21,52.7 28.57,53.34 19.68,53.34 17.78,51.44 11.43,51.44 11.43,48.9 15.88,48.9 17.14,47.62 17.14,21.59 18.16,20.57 19.68,20.57 19.68,19.05 18.41,19.05 18.41,15.88 16.51,15.88 16.51,12.06 34.29,12.06 34.92,11.43 34.92,7.62 34.29,6.99 32.38,6.99 31.75,6.35 31.75,1.91 36.83,1.91 36.83,13.97 23.5,13.97 22.86,14.61 22.86,19.05 19.68,22.23 19.68,38.73 19.05,39.37 19.05,48.9 20.32,50.16 29.21,50.16
!RST!  (via drill 0.5)
  Top 0.203: R1.1 52.07,20.88 S1.2 51.51,18.97 52.7,17.78 57.15,17.78 57.78,17.14 J11.5 | IC4.7 36.58,28.96 v36.83,29.21
  Bottom 0.203: v36.83,29.21 38.1,29.21 46.99,20.32 S1.2
+9V
  Top 0.203: R19.2 17.52,60.59 J5.2
  pour Top (isolate 0.203, rank 3): 17.14,60.96 17.14,59.05 24.77,59.05 25.4,59.69 29.97,59.69 29.97,57.78 30.99,57.78 30.99,60.96
A+
  Top 0.203: C25.2 19.32,18.41 R17.2 R16.1 14.97,16.14 14.61,16.51 IC7.3
A-
  Top 0.203: R10.2 13.34,22.49 13.71,22.12 R18.1 13.71,19.95 13.97,19.68 15.24,19.68 15.88,19.05 IC7.2
ADXL_SDO
  Top 0.203: IC8.12 14.54,33.32 R12.2
AGND  (via drill 0.5)
  other vias: 3.81,10.79 3.81,1.91 9.53,6.35
  pour Top (isolate 0.203, rank 2): 1.27,12.06 1.27,1.27 10.16,1.27 10.16,12.06
  pour Bottom (isolate 0.203, rank 2): 1.27,12.06 1.27,1.27 10.16,1.27 10.16,12.06
B_CSADC
  Top 0.203: R3.2 55.65,56.75 54.61,57.78 50.73,57.78 J3.7
B_CSHUM
  Top 0.203: R3.4 53.98,55.87 53.34,56.52 44.01,56.52 J3.3
B_CSPRS
  Top 0.203: R3.3 54.84,56.28 53.98,57.15 49.37,57.15 J3.6
B_LORA  (via drill 0.5)
  Top 0.203: R22.2 44.82,52.34 v44.45,52.7
  Bottom 0.203: v44.45,52.7 43.37,52.7 J13.3
B_MISO
  Top 0.203: J3.9 54.1,58.42 55.24,58.42 56.45,57.22 R3.1 56.97,56.4 D4.C
  Bottom 0.203: J3.9 52.83,59.18 52.07,58.42 48.26,58.42 46.83,56.99 J13.6
B_MOSI
  Top 0.203: J3.2 J13.2 37.47,53.88 R8.2 35.95,52.34 D9.C
B_SCK
  Top 0.203: R5.2 40.91,52.34 | 40.91,52.34 42.83,54.26 J13.4 | D8.C 41.29,51.95 40.91,52.34
  Bottom 0.203: J13.4 J3.4
BC
  Top 0.203: R13.2 43.81,5.08 41.48,2.75 D3.4
BOOT0
  Top 0.203: IC4.44 38.62,36.95 38.1,37.47 R26.1
BTN  (via drill 0.5)
  Top 0.203: S2.2 61.59,20.88 R7.1 54.98,23.23 v53.98,22.23 | IC4.2 35.85,31.46 v36.83,30.48
  Bottom 0.203: v36.83,30.48 38.1,30.48 46.35,22.23 v53.98,22.23
CSA0  (via drill 0.5)
  Top 0.203: IC3.1 44.08,42.28 v43.81,42.55 | IC4.43 39.12,37.72 36.83,40.01 v36.83,41.27
  Bottom 0.203: v36.83,41.27 38.1,42.55 v43.81,42.55
CSA1  (via drill 0.5)
  Top 0.203: IC4.42 39.62,38.48 v38.73,39.37 | v43.18,41.27 43.81,40.64 45.09,40.64 45.37,40.92 IC3.2
  Bottom 0.203: v38.73,39.37 40.64,41.27 v43.18,41.27
CSA2  (via drill 0.5)
  Top 0.203: IC4.25 47.41,26.46 48.26,27.3 v48.26,36.2 | IC3.3 46.02,40.3 45.72,40.01 v42.55,40.01
  Bottom 0.203: v42.55,40.01 45.72,40.01 46.35,40.64 48.26,40.64 48.9,40.01 48.9,36.83 v48.26,36.2
CSADC
  Top 0.203: IC3.10 48.62,49.25 50.8,51.44 53.98,51.44 55.65,53.1 R3.7
CSBHUM
  Top 0.203: IC3.12 47.31,50.49 49.53,52.7 52.7,52.7 54.05,54.05 R3.5
CSHUM
  Top 0.203: IC9.3 53.98,43.18 52.7,44.45 50.8,44.45 48.9,46.35 46.99,46.35 46.66,46.68 IC3.13
CSLAT
  Top 0.203: IC4.38 41.62,36.54 42.28,37.2 R6.1 42.28,38.47 43.18,39.37 46.35,39.37 46.66,39.68 IC3.4
CSLORA
  Top 0.203: IC3.14 46.02,50.24 R22.1
CSPRS
  Top 0.203: R3.6 54.84,53.58 53.34,52.07 50.16,52.07 47.97,49.87 IC3.11
CSSD  (via drill 0.5)
  Top 0.203: IC3.15 45.37,46.71 46.35,45.72 48.26,45.72 50.16,43.81 50.16,38.73 v55.24,33.66
  Bottom 0.203: v55.24,33.66 56.01,32.89 J4.2
DAC
  Top 0.203: IC4.14 37.12,21.25 33.02,17.14 26.67,17.14 25.4,18.41 C25.1 23.23,18.31
FB5
  Top 0.203: R11.2 28.2,55.51 27.57,54.88 | R10\.1 27.57,54.88 | IC5.5 28.77,53.68 27.57,54.88
GC
  Top 0.203: D3.6 40.44,6.14 40.01,6.58 R14.2
GND  (via drill 0.5, 0.6)
  Bottom 0.203: JP1.2 3.81,13.97
  Bottom 0.406: IC1.1 12.06,3.81
  other vias: 12.06,1.91 8.89,22.23 42.55,35.56 50.16,46.99 27.94,15.88 13.34,39.37 20.32,41.27 10.16,52.07 17.78,10.16 45.72,32.38 41.27,48.26 40.64,29.84 38.1,27.94 31.75,19.05 36.2,18.41 13.34,26.67
  pour Bottom (isolate 0.203, rank 4): 1.27,13.34 1.27,62.23 62.23,62.23 62.23,12.7 48.9,12.7 48.9,1.27 11.43,1.27 11.43,13.34
  pour Top (isolate 0.203, rank 4): 1.27,62.23 1.27,13.34 11.43,13.34 11.43,1.27 48.9,1.27 48.9,12.7 62.23,12.7 62.23,62.23
GPSBOOT
  Bottom 0.203: IC1.10 11.43,15.24 12.06,15.88 R4.1
GPSRX  (via drill 0.5)
  Top 0.203: IC4.22 41.12,23.02 43.18,20.95 43.18,19.05 v43.81,18.41
  Bottom 0.203: IC1.24 27.94,8.89 31.11,12.06 32.38,12.06 | v43.81,18.41 43.81,15.88 40.01,12.06 32.38,12.06 | R2.5 32.4,12.07 32.38,12.06
GPSTX  (via drill 0.5)
  Top 0.203: IC4.21 40.62,22.25 41.91,20.95 v41.91,19.68
  Bottom 0.203: v41.91,19.68 38.73,16.51 29.84,16.51 27.3,13.97 IC1.20
HXEN
  Top 0.203: R23.1 37.73,9.26 IC6.4 | 37.62,14.08 R23.1 | IC4.16 38.12,18.43 37.73,18.05 R23.1
LEDB
  Top 0.203: IC4.19 39.62,20.7 43.81,16.51 R13.1
LEDG
  Top 0.203: R14.1 40.01,17.78 38.62,19.16 IC4.17
LEDR
  Top 0.203: R15.1 41.91,17.14 39.12,19.93 IC4.18
LP1
  Top 0.203: IC7.1 17.14,19.32 R18.2 15.51,22.59 13.97,24.13 11.43,24.13 10.16,22.86 10.16,19.68 11.43,18.41 R27.1
LP2
  Top 0.203: R27.2 12.96,15.61 13.34,15.24 IC7.5 13.34,10.79 12.7,10.16 C39.1
LP-
  Top 0.203: IC7.6 14.61,10.43 R28.1
MISO  (via drill 0.5)
  Top 0.203: R3.8 56.45,50.09 55.24,48.9 IC9.5 55.8,47.07 56.52,46.35 v56.52,45.72 | IC4.40 40.62,42.56 40.01,43.18 v40.01,45.09
  Bottom 0.203: J4.7 56.3,38.32 55.88,38.73 55.88,41.27 56.52,41.91 v56.52,45.72 40.64,45.72 v40.01,45.09
MOSI  (via drill 0.5)
  Top 0.203: v40.01,31.75 40.12,31.86 IC4.41 40.12,41.8 37.47,44.45 R8.1
  Bottom 0.203: J4.3 56.23,33.94 55.24,34.92 43.81,34.92 43.18,34.29 40.76,34.29 40.12,33.66 40.12,31.86 v40.01,31.75
OSC32_IN
  Top 0.203: C8.1 32.12,36.56 31.43,35.88 Y1.1 31.43,32.07 32.54,30.96 IC4.3
OSC32_OUT
  Top 0.203: C9.1 27.57,36.56 28.26,35.88 Y1.4 28.26,33.97 31.77,30.46 IC4.4
OSC_IN
  Top 0.203: IC4.5 31,29.96 28.95,32.02 C7.1 27.68,32.02 25.65,34.04 Y2.1
OSC_OUT
  Top 0.203: IC4.6 31.36,29.46 28.31,26.41 C6.1 27.68,26.41 25.65,24.38 Y2.2
PG5
  Top 0.203: IC5.8 33.62,53.68 R9.1
PHOTO_GP2  (via drill 0.5)
  Top 0.203: D6.3 8.9,29.23 v8.26,28.57 8.26,22.86 5.17,19.78 J12.3 | 38.12,26.05 v38.73,26.67 37.62,25.55 IC4.15
  Bottom 0.203: v38.73,26.67 36.2,24.13 17.78,24.13 13.34,28.57 v8.26,28.57
PHOTO_GP4  (via drill 0.5)
  Top 0.203: D6.1 7.62,32.16 7.62,30.48 v7.3,30.16 7.08,29.94 J9.3 | v34.92,25.4 34.87,25.45 IC4.12
  Bottom 0.203: v34.92,25.4 18.41,25.4 13.88,29.94 7.53,29.94 v7.3,30.16
RC
  Top 0.203: R15.2 41.91,5.08 41.27,4.45 D3.5
RF_GPS
  Bottom 1.232: IC1.3 J7.SIG
RF_HX1
  Top 1.232: IC6.2 J6.SIG
RGND  (via drill 0.5)
  other vias: 51.44,3.81 60.33,3.81
  pour Top (isolate 0.203, rank 2): 62.23,1.27 50.16,1.27 50.16,11.43 62.23,11.43
  pour Bottom (isolate 0.203, rank 2): 50.16,11.43 50.16,1.27 62.23,1.27 62.23,11.43
RXA  (via drill 0.6)
  Bottom 0.203: R2.7 30.48,14.37 | 30.48,14.37 28.98,14.37 27.3,12.7 IC1.21 | v30.48,15.24 30.48,14.37
SCK  (via drill 0.5)
  Top 0.203: v55.24,43.81 IC9.4 | IC4.39 41.12,43.66 v41.27,43.81 41.27,46.35 40.01,47.62 R5.1
  Bottom 0.203: J4.5 55.98,36.09 54.61,37.47 54.61,43.18 v55.24,43.81 v41.27,43.81
SCL  (via drill 0.5)
  Top 0.203: J1.4 J2.4 13.21,54.09 D7.C | IC4.45 38.12,35.67 v37.59,36.2 | v17.14,36.83 IC8.14
  Bottom 0.203: v37.59,36.2 17.78,36.2 v17.14,36.83 16.51,37.47 16.51,49.53 12.38,53.66 | J2.4 11.43,54.61 12.38,53.66 | R21.2 12.7,53.98 12.38,53.66
SDA  (via drill 0.5)
  Top 0.203: J1.3 J2.3 10.79,53.98 12.06,53.98 13.34,52.7 D5.C | IC4.46 37.62,32.23 v38.1,31.75 | IC8.13 15.34,34.83 v15.88,34.29
  Bottom 0.203: v38.1,31.75 38.1,33.66 36.83,34.92 16.51,34.92 | 16.51,34.92 v15.88,34.29 | J2.3 8.89,55.24 10.16,53.98 | 10.16,53.98 15.24,48.9 15.24,36.2 16.51,34.92 | R29.2 9.53,53.34 10.16,53.98
SW5
  pour Top (isolate 0.203, rank 3, no thermals): 30.73,53.98 30.73,50.55 31.11,50.16 32.26,50.16 32.26,52.58 31.11,52.58 31.11,53.98
SWCLK  (via drill 0.5)
  Top 0.203: IC4.37 42.12,31.96 v41.91,31.75 | J11.2 v50.16,23.5
  Bottom 0.203: v41.91,31.75 41.91,27.94 46.35,23.5 v50.16,23.5
SWDIO  (via drill 0.5)
  Top 0.203: IC4.34 45.88,30.96 v46.35,30.48
  Bottom 0.203: v46.35,30.48 50.16,26.67 51.44,26.67 56.52,21.59 56.52,16.89 J11.4
TEMPB  (via drill 0.5)
  Top 0.203: D6.6 v7.61,34.91 7.62,34.92 7.62,39.37 6.89,40.1 J10.3 | IC4.11 33.95,26.96 v33.66,26.67
  Bottom 0.203: v33.66,26.67 19.05,26.67 14.61,31.11 11.4,31.11 v7.61,34.91
TEMPG  (via drill 0.5)
  Top 0.203: J8.3 4.99,50.26 5.71,49.53 6.99,49.53 8.9,47.61 8.9,36.83 v8.9,36.2 D6.4 | IC4.10 36.67,27.46 v36.83,27.3
  Bottom 0.203: v36.83,27.3 36.2,27.94 19.68,27.94 15.24,32.38 12.71,32.38 v8.9,36.2
TXA  (via drill 0.6)
  Bottom 0.203: R2.6 30.08,13.57 v27.94,11.43 26.67,10.16 IC1.23
TXD
  Top 0.203: IC6.7 16.51,8.89 16.14,9.26 R28.2 15.88,10.43 IC7.7
VCORE
  Top 0.406: IC9.1 51.44,39.63 C28.1
VDDA
  pour Top (isolate 0.203, rank 2): 32.38,22.86 29.21,22.86 29.21,24.77 32.46,28.02 35.56,28.02 35.56,27.3 33.02,27.3 32.38,26.67
VDIV  (via drill 0.5)
  Top 0.203: R19.1 15.24,57.78 16.88,56.15 R20.2 17.78,53.71 v17.78,52.07 | IC4.13 36.62,22.02 32.38,17.78 27.3,17.78 25.4,19.68 22.86,19.68 19.68,22.86 19.68,37.47 v20.32,38.1
  Bottom 0.203: v20.32,38.1 20.32,39.37 17.78,41.91 v17.78,52.07
VS  (via drill 0.5)
  Top 0.305: 8.26,33.02 9.53,33.02 10.16,33.66 10.16,36.2 10.79,36.83 IC8.7
  Top 0.406: IC9.8 51.44,48.9 | 51.44,48.9 v50.8,49.53 | 51.44,48.9 51.8,48.9 C29.1 | IC8.7 11.34,36.93 IC8.6 11.34,39.65 C23.1 C24.1 15.34,39.65 IC8.1
  Bottom 0.406: v50.8,49.53 54.83,53.56 J3.10
  pour Top (rank 2): 9.53,14.61 1.91,14.61 1.27,15.24 1.27,52.7 1.91,53.34 8.89,53.34 8.89,50.8 8.26,50.8 7.62,51.44 2.54,51.44 1.91,50.8 1.91,47.62 2.54,46.99 6.35,46.99 6.35,45.72 2.54,45.72 1.91,45.09 1.91,37.47 2.54,36.83 6.99,36.83 6.99,33.66 8.26,33.66 8.26,33.02 6.35,33.02 3.81,35.56 2.54,35.56 1.91,34.92 1.91,27.3 2.54,26.67 6.35,26.67 6.35,25.4 2.54,25.4 1.91,24.77 1.91,17.14 2.54,16.51 9.53,16.51
  pour Bottom (isolate 0.203, rank 2): 5.08,46.99 5.08,45.72 1.27,45.72 1.27,62.23 55.88,62.23 55.88,58.42 50.16,58.42 50.16,60.33 49.53,60.96 3.17,60.96 2.54,60.33 2.54,47.62 3.17,46.99
XRESET
  Bottom 0.203: R24.2 10.16,17.14 9.53,16.51 IC1.11
XSTBY  (via drill 0.5)
  Top 0.203: IC4.20 40.12,21.48 v40.64,20.95
  Bottom 0.203: IC1.16 28.2,19.05 R25.2 39.74,20.05 v40.64,20.95

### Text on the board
tPlace: I2C | 9V | BOTTOM | + | LORA | TEMP / GPS | TEMP / BATT | SD | RST | BTN | PHOTO / GP4 | RXA | PHOTO / GP2 | TXA | GPS | RF | THIS SIDE UP
bPlace: Microsoft Maker Garage | HAB Project | Telemetry Rev 3 | Contact / ~STCARLSO / 301 956 5041 | PROGRAM

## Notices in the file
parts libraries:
SparkFun-Aesthetics: Licensing: Creative Commons ShareAlike 4.0 International - https://creativecommons.org/licenses/by-sa/4.0
SparkFun-Aesthetics: Released under the Creative Commons Attribution Share-Alike 4.0 License
SparkFun-Aesthetics: https://creativecommons.org/licenses/by-sa/4.0
